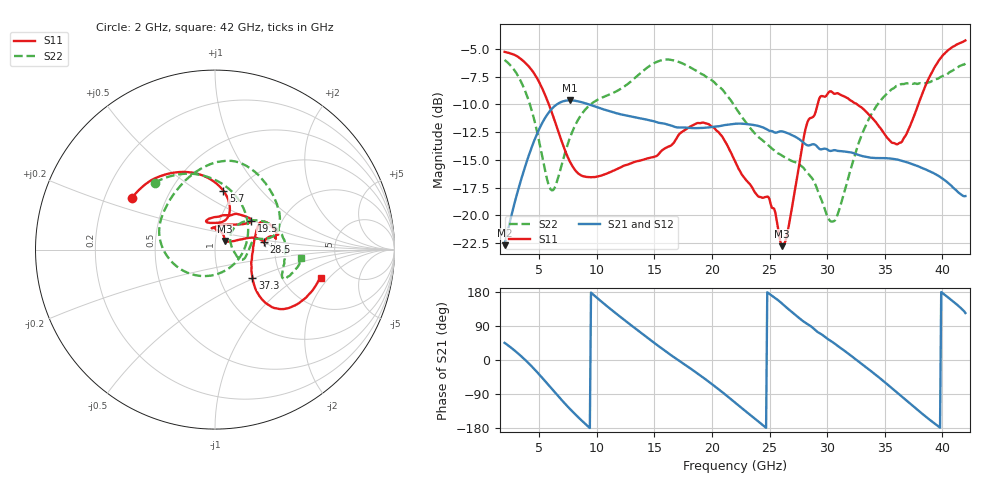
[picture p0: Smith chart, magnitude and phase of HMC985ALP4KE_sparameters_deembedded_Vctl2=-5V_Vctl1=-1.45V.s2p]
!s2p File: Measurements: S11, S21, S12, S22
# GHz S dB R 50.0
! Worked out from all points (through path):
!   401 points, 2 GHz to 42 GHz, reference 50 ohm
!   highest |S21| = -9.64 dB at 7.7 GHz (marker M1); lowest = -22.7 dB at 2 GHz (marker M2)
!   lowest |S11| = -22.8 dB at 26.1 GHz (marker M3), VSWR 1.16, Z = 55.5 + j5.38 ohm
!   |S11| at or under -10 dB: 5.84 GHz to 29.17 GHz (23.33 GHz wide, 133 % of centre); 32.61 GHz to 37.91 GHz (5.303 GHz wide, 15 % of centre)
!   |S22| runs from -20.6 to -6.0 dB; largest |S21 - S12| = 0.00037
!   S11 on the Smith chart (normalised r, x): 2 GHz: 0.32, +0.26; 5.7 GHz: 0.88, +0.64; 19.5 GHz: 1.41, +0.49; 28.5 GHz: 1.73, +0.16; 37.3 GHz: 1.43, -0.48; 42 GHz: 3.25, -1.67
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2  -5.27 148.3  -22.70 45.3  -22.71 45.3  -6.00 132.1
3.6  -6.07 121.8  -16.20 5.6  -16.21 5.6  -8.35 88.0
4.7  -7.44 100.8  -12.94 -28.0  -12.94 -28.0  -11.93 46.0
5.7  -9.63 81.8  -10.92 -62.2  -10.93 -62.2  -16.80 -17.7
6.3  -11.33 73.1  -10.19 -83.3  -10.20 -83.2  -17.61 -72.8
7.7  -15.22 70.8  -9.64 -130.0  -9.64 -130.0  -12.93 -153.0
8.7  -16.43 82.3  -9.80 -160.0  -9.81 -160.0  -10.86 -179.4
10.2  -16.47 98.7  -10.31 159.4  -10.32 159.4  -9.51 157.9
12.1  -15.66 107.5  -10.90 112.6  -10.90 112.6  -8.59 133.1
15.4  -14.45 80.9  -11.66 36.0  -11.66 36.0  -6.10 84.5
19.5  -11.72 38.5  -12.09 -52.2  -12.10 -52.2  -7.52 33.6
22  -15.11 52.6  -11.74 -112.2  -11.75 -112.2  -10.20 12.0
24.9  -18.34 93.6  -12.34 176.4  -12.34 176.4  -13.69 10.0
26.1  -22.77 41.6  -12.43 148.4  -12.44 148.4  -14.62 -2.6
28.5  -11.25 8.9  -13.68 90.9  -13.68 91.0  -16.43 -20.7
28.7  -11.18 8.3  -13.60 86.3  -13.61 86.3  -16.66 -20.2
30.6  -9.04 14.7  -14.12 44.3  -14.12 44.4  -20.50 21.8
33.2  -10.48 30.9  -14.69 -15.0  -14.70 -15.0  -12.26 41.4
35.4  -13.21 8.4  -14.87 -68.7  -14.87 -68.7  -8.84 18.9
37.3  -11.69 -36.9  -15.35 -117.6  -15.35 -117.6  -8.12 -2.2
39.7  -6.04 -41.7  -16.46 -176.3  -16.46 -176.2  -7.63 -23.3
42  -4.24 -15.1  -18.26 123.9  -18.26 123.9  -6.30 -5.8
